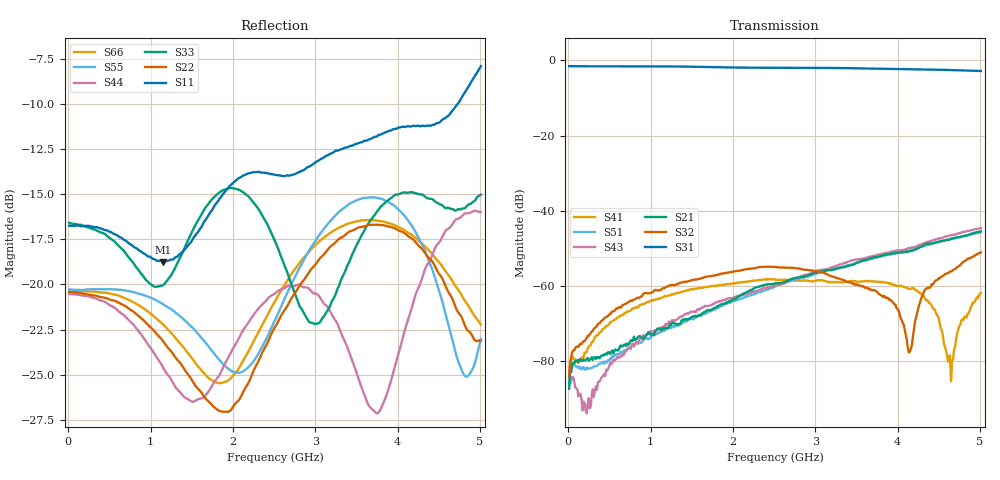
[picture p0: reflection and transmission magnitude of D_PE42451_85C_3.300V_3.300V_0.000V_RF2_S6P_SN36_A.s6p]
! Device ID: PE42451
! Serial: 36
! Insertion: A
! Temp: 85C
! VDD: 3.300
! Control_Hi: 100.000
! Control_Lo: 0.000
! Logic State: RF2
! Port 1: RFC
! Port 2: RF1
! Port 3: RF2
! Port 4: RF3
! Port 5: RF4
! Port 6: RF5
! V1 = 0.00
! V2 = 3.30
! V3 = 0.00
! V4 = 0.00
! IDD: 1.757800e-05
#  Hz  S  RI  R  50
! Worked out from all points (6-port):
!   401 points, 10 MHz to 5.01 GHz, reference 50 ohm
!   strongest paths, dB at 10 MHz, 1.26 GHz, 2.51 GHz, 3.76 GHz, 5.01 GHz:
!     S31: -1.5, -1.6, -2.0, -2.2, -2.8
!     S32: -84.0, -59.6, -54.9, -61.8, -51.0
!     S21: -87.3, -69.7, -59.3, -52.2, -45.5
!     S43: -85.4, -69.0, -59.8, -51.7, -44.6
!     S51: -85.4, -70.9, -60.1, -52.3, -45.7
!     S41: -84.9, -62.1, -58.2, -58.9, -61.8
!   lowest |S11| = -18.8 dB at 1.147 GHz (marker M1), VSWR 1.26, Z = 57.8 - j9.72 ohm
!   |S11| at or under -10 dB: start of sweep to 4.73 GHz
